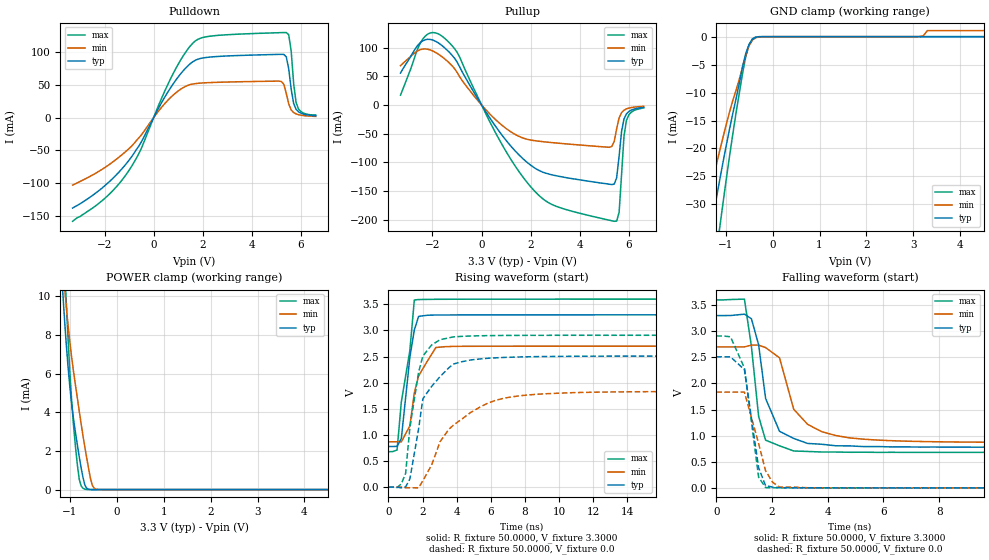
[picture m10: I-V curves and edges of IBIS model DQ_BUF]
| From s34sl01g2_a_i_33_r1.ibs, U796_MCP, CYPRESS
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|   Model DQ_BUF
[Model]  DQ_BUF
Model_type I/O
Vinl =   0.6600V | Vinl = Vio*0.3
Vinh =   2.6400V | Vinh = Vio*0.8
Vmeas =  1.6500V | Vmeas = Vio*0.5
Cref =   30.0000pF
C_comp   3.37pF   3.03pF   4.30pF
[Temperature Range]   25.0000   85.0000   -40.0000
[Pullup Reference]   3.3000V   2.7000V   3.6000V
[Pulldown Reference]   0.0V   0.0V   0.0V
[POWER Clamp Reference]   3.3000V   2.7000V   3.6000V
[GND Clamp Reference]   0.0V   0.0V   0.0V
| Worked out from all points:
|   slope of the pulldown table from 0 to 0.495 V, typ, clamps not added: 14.7 ohm
|   slope of the pullup table from 0 to 0.495 V, typ, clamps not added: 15.2 ohm
|   GND clamp passes 1 mA (typ) near -0.47 V on its own axis
|   POWER clamp passes 1 mA (typ) near -0.75 V on its own axis
|   rising waveform, R_fixture 50.0000, V_fixture 3.3000: 20-80 % time 541ps typ, 853ps min, 707ps max; typ from 0.779 V to 3.3 V
|   rising waveform, R_fixture 50.0000, V_fixture 0.0: 20-80 % time 1.3ns typ, 2.57ns min, 770ps max; typ from 0 V to 2.51 V
|   falling waveform, R_fixture 50.0000, V_fixture 3.3000: 20-80 % time 621ps typ, 895ps min, 401ps max; typ from 3.3 V to 0.779 V
|   falling waveform, R_fixture 50.0000, V_fixture 0.0: 20-80 % time 409ps typ, 551ps min, 443ps max; typ from 2.51 V to 0 V
[Pulldown]
|Voltage   I(typ)   I(min)   I(max)
-3.3V     -137.8mA   -102.9mA   -158mA
-1.1V     -69.56mA   -50.51mA   -85.71mA
900mV     56.9mA     37.59mA    74.42mA
1.8V      88.84mA    52.12mA    119.1mA
5.1V      96.17mA    55.45mA    129.2mA
5.4V      92.37mA    36.76mA    129.4mA
5.5V      73.99mA    20.64mA    126mA
5.6V      43.01mA    11.6mA     101.1mA
5.7V      21.45mA    7.52mA     51.5mA
5.8V      12.51mA    5.49mA     22.8mA
6V        6.58mA     3.52mA     8.9mA
6.6V      2.7mA      1.7mA      4mA
[Pullup]
|Voltage   I(typ)   I(min)   I(max)
-3.3V     55.55mA    68.5mA     17mA
-2.4V     111.6mA    97.37mA    114.5mA
-1.7V     106.3mA    86.73mA    122.4mA
-1V       75mA       56.95mA    92.01mA
700mV     -44.99mA   -30.62mA   -58.83mA
2.2V      -110.8mA   -62.44mA   -151.9mA
5.4V      -138mA     -63.5mA    -202.7mA
5.5V      -126.9mA   -41.6mA    -202.4mA
5.6V      -88.99mA   -22.61mA   -187mA
5.8V      -24.3mA    -9.1mA     -53.71mA
5.9V      -15.49mA   -6.82mA    -26.56mA
6.6V      -4.3mA     -2.4mA     -5mA
[GND_clamp]
|Voltage   I(typ)   I(min)   I(max)
-3.3V     -993.2mA   -397.9mA   -1.959A
-1.48V    -42.63mA   -33.34mA   -57.88mA
-1.34V    -35.68mA   -28.07mA   -48.21mA
-1.27V    -32.3mA    -25.5mA    -43.51mA
-1.13V    -25.77mA   -20.52mA   -34.37mA
-780mV    -11.16mA   -9.617mA   -13.71mA
-570mV    -2.965mA   -3.308mA   -3.505mA
-500mV    -1.356mA   -1.606mA   -1.413mA
-360mV    -117uA     -187.5uA   -58.29uA
3.14V     756.3pA    21.25uA    371.5pA
3.3V      808.9pA    1.086mA    399pA
6.6V      808.9pA    1.086mA    399pA
[POWER_clamp]
|Voltage   I(typ)   I(min)   I(max)
-3.28V    954.7mA    449.2mA    1.77A
-1.16V    10.56mA    11.89mA    14.41mA
-1.12V    9.036mA    10.68mA    12.1mA
-1.08V    7.645mA    9.57mA     9.906mA
-1V       5.324mA    7.642mA    6.093mA
-960mV    4.398mA    6.817mA    4.554mA
-880mV    2.947mA    5.402mA    2.224mA
-800mV    1.702mA    4.066mA    543.8uA
-680mV    237.8uA    2.197mA    22.81uA
-520mV    1.459uA    215.4uA    122.7nA
-400mV    29.81nA    6.336uA    1.481nA
6.6V      0A         0A         0A
[Ramp]
| variable   typ   min   max
dV/dt_r  1.5058/1.2228n   1.0995/2.2827n   1.7450/0.6812n
dV/dt_f  1.5126/0.6688n   1.0985/1.1920n   1.7520/0.5003n
R_load = 50.0000
[Rising Waveform]
R_fixture= 50.0000
V_fixture= 3.3000
V_fixture_min= 2.7000
V_fixture_max= 3.6000
|time   V(typ)   V(min)   V(max)
0s        778.8mV    869mV      679.7mV
250ps     778.6mV    868.8mV    680.2mV
510ps     779.9mV    868.4mV    711mV
760ps     934.2mV    867.2mV    1.634V
1.26ns    2.489V     1.175V     2.622V
1.52ns    3.01V      1.809V     3.584V
1.77ns    3.269V     2.129V     3.592V
2.78ns    3.296V     2.674V     3.597V
4.29ns    3.298V     2.697V     3.598V
25ns      3.3V       2.7V       3.6V
[Rising Waveform]
R_fixture= 50.0000
V_fixture= 0.0
V_fixture_min= 0.0
V_fixture_max= 0.0
|time   V(typ)   V(min)   V(max)
0s        179.1uV    275.7uV    124.5uV
510ps     -214.6uV   30.69uV    -8.824mV
1.01ns    4.965mV    -11.24mV   263.5mV
1.26ns    157.6mV    -11.24mV   1.141V
1.77ns    1.115V     -13.56mV   2.203V
2.02ns    1.691V     122.4mV    2.51V
3.03ns    2.118V     871.1mV    2.824V
4.8ns     2.434V     1.426V     2.894V
7.32ns    2.489V     1.733V     2.905V
25ns      2.51V      1.833V     2.908V
[Falling Waveform]
R_fixture= 50.0000
V_fixture= 3.3000
V_fixture_min= 2.7000
V_fixture_max= 3.6000
|time   V(typ)   V(min)   V(max)
0s        3.3V       2.7V       3.6V
1.01ns    3.327V     2.7V       3.615V
1.26ns    3.24V      2.733V     2.712V
1.52ns    2.739V     2.733V     1.368V
1.77ns    1.712V     2.686V     913.5mV
2.27ns    1.084V     2.49V      805.1mV
2.78ns    946.3mV    1.504V     706.1mV
3.79ns    834.8mV    1.075V     686.6mV
5.81ns    791mV      914mV      679.9mV
25ns      778.8mV    869mV      680mV
[Falling Waveform]
R_fixture= 50.0000
V_fixture= 0.0
V_fixture_min= 0.0
V_fixture_max= 0.0
|time   V(typ)   V(min)   V(max)
0s        2.51V      1.833V     2.909V
510ps     2.509V     1.833V     2.893V
1.01ns    2.263V     1.833V     2.297V
1.52ns    383mV      848.1mV    202.8mV
1.77ns    42.68mV    326.9mV    5.316mV
2.02ns    15.1mV     107mV      2.515mV
2.27ns    3.928mV    13.8mV     1.233mV
4.29ns    258.3uV    785.1uV    193.1uV
25ns      177uV      273.8uV    124.1uV
